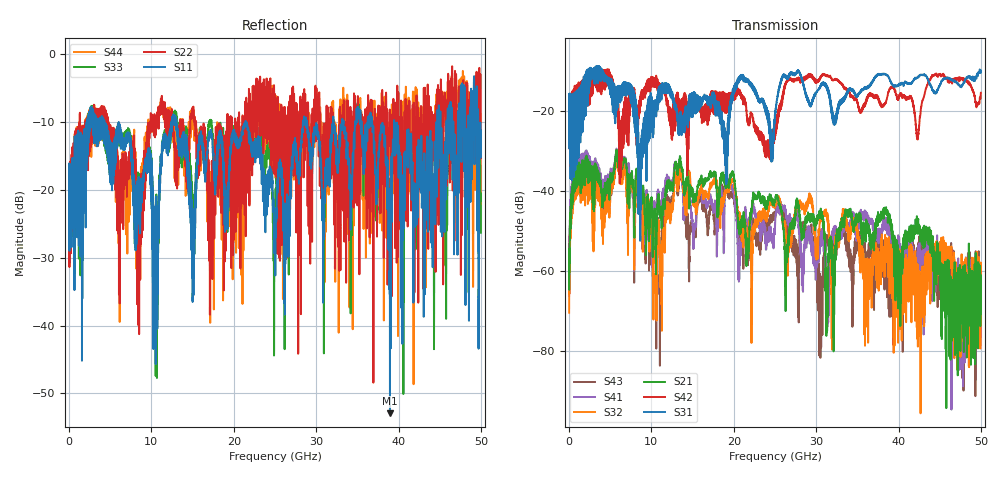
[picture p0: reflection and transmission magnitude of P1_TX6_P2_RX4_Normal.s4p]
!Keysight Technologies,N5225B,MY57041031,A.13.20.10
!Date: Friday, May 31, 2019 11:33:44
!Correction: S11(Full 4 Port(1,2,3,4))
!S12(Full 4 Port(1,2,3,4))
!S13(Full 4 Port(1,2,3,4))
!S14(Full 4 Port(1,2,3,4))
!S21(Full 4 Port(1,2,3,4))
!S22(Full 4 Port(1,2,3,4))
!S23(Full 4 Port(1,2,3,4))
!S24(Full 4 Port(1,2,3,4))
!S31(Full 4 Port(1,2,3,4))
!S32(Full 4 Port(1,2,3,4))
!S33(Full 4 Port(1,2,3,4))
!S34(Full 4 Port(1,2,3,4))
!S41(Full 4 Port(1,2,3,4))
!S42(Full 4 Port(1,2,3,4))
!S43(Full 4 Port(1,2,3,4))
!S44(Full 4 Port(1,2,3,4))
!S4P File: Measurements: <S11,S12,S13,S14>,
!<S21,S22,S23,S24>,
!<S31,S32,S33,S34>,
!<S41,S42,S43,S44>:
# Hz S  dB  R 50.0
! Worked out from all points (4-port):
!   5000 points, 10 MHz to 50 GHz, reference 50 ohm
!   strongest paths, dB at 10 MHz, 12.51 GHz, 25.01 GHz, 37.51 GHz, 50 GHz:
!     S31: -19.4, -15.5, -21.6, -10.8, -9.9
!     S42: -19.6, -27.2, -23.9, -16.7, -15.4
!     S21: -58.2, -38.4, -42.4, -45.2, -62.9
!     S32: -70.4, -43.5, -43.5, -58.0, -59.3
!     S41: -66.1, -38.0, -49.1, -50.6, -76.6
!     S43: -57.3, -42.2, -46.2, -50.0, -64.1
!   lowest |S11| = -52.9 dB at 38.96 GHz (marker M1), VSWR 1.00, Z = 50.2 + j0.118 ohm
!   |S11| at or under -10 dB: 4.286 GHz to 12.47 GHz (8.179 GHz wide, 97.7 % of centre); 13.02 GHz to 21.43 GHz (8.403 GHz wide, 48.8 % of centre); 21.46 GHz to 28.42 GHz (6.96 GHz wide, 27.9 % of centre)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
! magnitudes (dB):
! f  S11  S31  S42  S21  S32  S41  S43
! 10 MHz  -19.4  -19.4  -19.6  -58.2  -70.4  -66.1  -57.3
! 910 MHz  -20.2  -20.7  -19.8  -33.9  -35.8  -31.6  -33.6
! 5.91 GHz  -11.9  -16.9  -21.3  -31.0  -31.8  -31.0  -31.5
! 11.22 GHz  -15.4  -17.2  -13.3  -45.4  -55.7  -44.8  -60.5
! 13.57 GHz  -12.9  -23.1  -19.8  -33.0  -34.8  -34.6  -35.6
! 38.96 GHz  -52.9  -12.3  -14.5  -47.4  -55.7  -50.0  -60.5
! 50 GHz  -11.3  -9.9  -15.4  -62.9  -59.3  -76.6  -64.1
